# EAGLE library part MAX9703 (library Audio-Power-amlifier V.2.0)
The MAX9703 mono class D audio power amplifiers provide class AB amplifier performance with class D efficiency, conserving board space and eliminating the need for a bulky heatsink. Using a class D architecture, these devices deliver up to 15W while offering up to 78% efficiency. Proprietary and patent-protected modulation and switching schemes render the traditional class D output filter unnecessary.
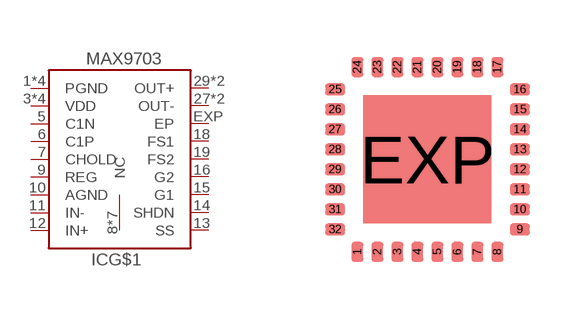
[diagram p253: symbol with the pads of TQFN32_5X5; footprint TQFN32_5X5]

Designator prefix IC; gates G$1=MAX9703 G$2=NC

## MAX9703  [TQFN32_5X5]
1  G$1:PGND  pwr
2  G$1:PGND  pwr
3  G$1:VDD  pwr
4  G$1:VDD  pwr
5  G$1:C1N
6  G$1:C1P
7  G$1:CHOLD
8  G$2:NC  nc
9  G$1:REG  out
10  G$1:AGND  pwr
11  G$1:IN-  in
12  G$1:IN+  in
13  G$1:SS
14  G$1:SHDN
15  G$1:G1  in
16  G$1:G2  in
17  G$2:NC  nc
18  G$1:FS1  in
19  G$1:FS2  in
20  G$2:NC  nc
21  G$1:VDD  pwr
22  G$1:VDD  pwr
23  G$1:PGND  pwr
24  G$1:PGND  pwr
25  G$2:NC  nc
26  G$2:NC  nc
27  G$1:OUT-  out
28  G$1:OUT-  out
29  G$1:OUT+  out
30  G$1:OUT+  out
31  G$2:NC  nc
32  G$2:NC  nc
EXP  G$1:EP  pwr

## Footprint TQFN32_5X5 (pad centres in mm)
TQFN32-5x5x0,8mm. Source: www.maxim-ic.com/packages
smd 0.3 x 0.5: 1 -1.75,-2.31; 2 -1.25,-2.31; 3 -0.75,-2.31; 4 -0.25,-2.31; 5 0.25,-2.31; 6 0.75,-2.31; 7 1.25,-2.31; 8 1.75,-2.31; 17 1.75,2.31; 18 1.25,2.31; 19 0.75,2.31; 20 0.25,2.31; 21 -0.25,2.31; 22 -0.75,2.31; 23 -1.25,2.31; 24 -1.75,2.31
smd 0.5 x 0.3: 9 2.31,-1.75; 10 2.31,-1.25; 11 2.31,-0.75; 12 2.31,-0.25; 13 2.31,0.25; 14 2.31,0.75; 15 2.31,1.25; 16 2.31,1.75; 25 -2.31,1.75; 26 -2.31,1.25; 27 -2.31,0.75; 28 -2.31,0.25; 29 -2.31,-0.25; 30 -2.31,-0.75; 31 -2.31,-1.25; 32 -2.31,-1.75
smd 3.2 x 3.2: EXP 0,0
